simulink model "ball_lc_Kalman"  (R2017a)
settings: Solver=ode45  StartTime=0.0  StopTime=10.0  RelTol=1e-3
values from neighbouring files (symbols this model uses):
  d = 0.03    [codigo_control_ss.m]    (also in codigo_control.m; codigo_control_simulacion.m)
  g = -9.8    [codigo_control_ss.m]    (also in codigo_control.m; codigo_control_simulacion.m)
  J = 5.1984e-5    (= 5.1984e-05)    [codigo_control_ss.m]    (also in codigo_control.m; codigo_control_simulacion.m)
  K = place(A,B,[p1,p2])    [codigo_control_ss.m]    (also in rscale.m = k; codigo_control_simulacion.m)
  L = 0.43    [codigo_control_ss.m]    (also in codigo_control.m; codigo_control_simulacion.m)
  m = 0.16    [codigo_control_ss.m]    (also in codigo_control.m; codigo_control_simulacion.m)
  Nbar = rscale(ball_ss,K)    [codigo_control_ss.m]    (also in rscale.m = Nu + K*Nx; codigo_control_simulacion.m)
  R = 0.0285    [codigo_control_ss.m]    (also in codigo_control.m; codigo_control_simulacion.m)
undefined symbols (not defined in the file or in its folder): Continuous, Time
libraries: ctrlSharedLib x1

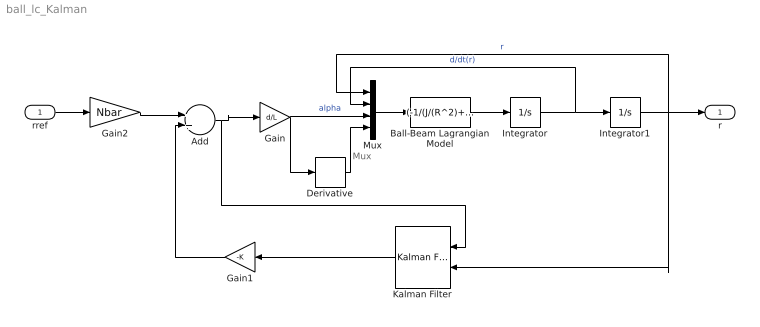
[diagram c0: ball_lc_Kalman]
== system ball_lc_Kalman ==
  note: Mux
  rref : Inport
  Add : Sum
  Ball-Beam Lagrangian Model : Fcn  Expr=(-1/(J/(R^2)+m))*(m*g*sin(u[3])-m*u[1]*(u[4])^2)
  Derivative : Derivative
  Gain : Gain  Gain=d/L
  Gain1 : Gain  Gain=-K  Multiplication=Matrix(K*u) (u vector)
  Gain2 : Gain  Gain=Nbar
  Integrator : Integrator
  Integrator1 : Integrator
  Kalman Filter : ctrlSharedLib/Kalman Filter  TimeDomain=Continuous-Time  UseCurrentEstimator=on  ModelSource=LTI State-Space Variable  ModelSourceVariable=ball_ss  A=0.95  B=1  C=1  D=0  NumberOfStates=1  NumberOfInputs=1  NumberOfOutputs=1  InitialEstimateSource=Dialog  X0=0  P0=10  UseK=off  UseGH=off  NumberOfProcessNoiseInputs=1  G=1  TimeInvariantG=on  H=0  TimeInvariantH=on  Q=0.05  TimeInvariantQ=on  R=1  TimeInvariantR=on  N=0  TimeInvariantN=on  AddInputPort=on  AddEnablePort=off  OutputEstimatedY=off  OutputP=off  Ts=-1
  Mux : Mux
  r : Outport
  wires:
  Integrator/1 -> Mux/2, Integrator1/1  "d/dt(r)"
  Integrator1/1 -> Kalman Filter/2, Mux/1, r/1  "r"
  Ball-Beam Lagrangian Model/1 -> Integrator/1
  Mux/1 -> Ball-Beam Lagrangian Model/1
  Gain/1 -> Derivative/1, Mux/3  "alpha"
  Derivative/1 -> Mux/4
  Kalman Filter/1 -> Gain1/1
  Gain1/1 -> Add/2
  Add/1 -> Kalman Filter/1, Gain/1
  Gain2/1 -> Add/1
  rref/1 -> Gain2/1
